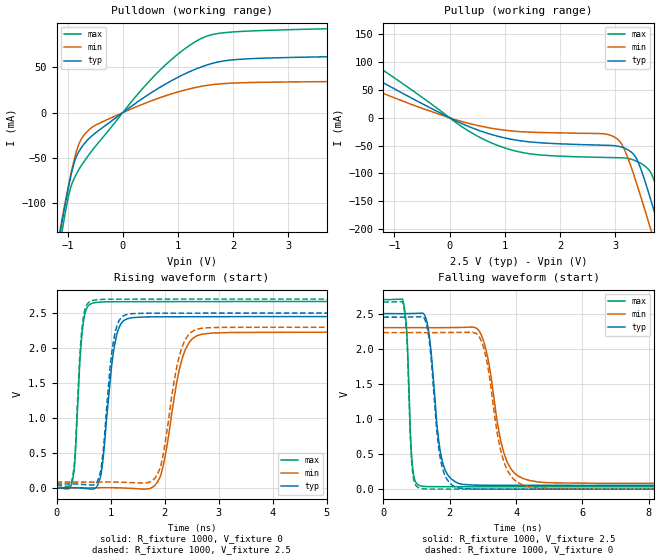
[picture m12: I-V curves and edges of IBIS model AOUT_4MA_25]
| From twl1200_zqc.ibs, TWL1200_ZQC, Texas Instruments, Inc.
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[Model]   AOUT_4MA_25
Model_type  Output
Vref =   2.5
Rref =   1M
Cref =   15p
Vmeas =   1.25
| variable   typ   min   max
C_comp   3.40pF   2.49pF   4.51pF
| C_pullup   3.64pF   2.49pF   4.51pF
| C_pulldown   3.15pF   2.72pF   3.73pF
[Temperature Range]   40   100   -40
| Ambient temperature   25   85   -40
[Voltage range]   2.5   2.3   2.7
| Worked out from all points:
|   slope of the pulldown table from 0 to 0.375 V, typ, clamps not added: 23.1 ohm
|   slope of the pullup table from 0 to 0.375 V, typ, clamps not added: 22.2 ohm
|   rising waveform, R_fixture 1000, V_fixture 0: 20-80 % time 186ps typ, 294ps min, 112ps max; typ from 0 V to 2.45 V
|   falling waveform, R_fixture 1000, V_fixture 2.5: 20-80 % time 289ps typ, 475ps min, 126ps max; typ from 2.5 V to 0.054 V
|   rising waveform, R_fixture 1000, V_fixture 2.5: 20-80 % time 171ps typ, 278ps min, 109ps max; typ from 0.054 V to 2.5 V
|   falling waveform, R_fixture 1000, V_fixture 0: 20-80 % time 278ps typ, 462ps min, 122ps max; typ from 2.45 V to 0 V
[Pulldown]
| AOUT_4MA_25
|   Voltage   I(typ)   I(min)   I(max)
-2.5V     -642.6mA   -610.7mA   -690.5mA
-1.15V    -137.8mA   -133.6mA   -149.9mA
-1.11V    -123.9mA   -120.4mA   -134.9mA
-1.085V   -115.3mA   -112.3mA   -125.8mA
-970mV    -78.33mA   -76.64mA   -88.69mA
-875mV    -54.32mA   -50.76mA   -71.95mA
-770mV    -40.49mA   -31.37mA   -60.2mA
-610mV    -28.5mA    -18.85mA   -46.14mA
575mV     24.18mA    14.3mA     40.68mA
1.41V     50.08mA    28.8mA     81.33mA
2.24V     59.27mA    33.09mA    89.82mA
5V        62.72mA    34.67mA    94.24mA
[Pullup]
| AOUT_4MA_25
|   Voltage   I(typ)   I(min)   I(max)
-2.5V     130mA      93.97mA    163.5mA
-430mV    21.91mA    14.65mA    31.96mA
770mV     -30.37mA   -19.01mA   -45.69mA
1.535V    -44.12mA   -26.1mA    -65.78mA
2.94V     -49.86mA   -32.46mA   -71.64mA
3.125V    -52.97mA   -48.42mA   -72.03mA
3.345V    -66.91mA   -104.7mA   -76.4mA
3.47V     -93.2mA    -143.6mA   -82.2mA
3.64V     -145.6mA   -199.1mA   -97.66mA
3.795V    -198.1mA   -251.1mA   -140.1mA
3.95V     -252.3mA   -304mA     -194.5mA
5V        -635.9mA   -673.3mA   -595.2mA
[Ramp]
| AOUT_4MA_25
| variable   typ   min   max
dV/dt_r   1.48/2.02E-10   1.35/3.05E-10   1.61/1.19E-10
dV/dt_f   1.47/2.94E-10   1.34/4.85E-10   1.60/1.27E-10
R_load = 1000
[Rising Waveform]
| AOUT_4MA_25
R_fixture =   1000
C_fixture =   0
L_fixture =   0
V_fixture =   0
V_fixture_min = 0
V_fixture_max = 0
|   Time   V(typ)   V(min)   V(max)
0s        9.079nV    37.27nV    970.3pV
310ps     1.537mV    -21.75uV   167.8mV
535ps     -9.551mV   -44.8uV    2.52V
820ps     179.2mV    1.28mV     2.657V
970ps     1.341V     1.868mV    2.661V
1.255ns   2.397V     -3.227mV   2.662V
1.92ns    2.446V     163.6mV    2.663V
2.46ns    2.447V     2.086V     2.664V
3.25ns    2.449V     2.222V     2.664V
238.2ns   2.45V      2.23V      2.665V
[Falling Waveform]
| AOUT_4MA_25
R_fixture =   1000
C_fixture =   0
L_fixture =   0
V_fixture =   2.5
V_fixture_min = 2.3
V_fixture_max = 2.7
|   Time   V(typ)   V(min)   V(max)
0s        2.5V       2.3V       2.7V
590ps     2.499V     2.3V       2.686V
705ps     2.5V       2.3V       2.232V
895ps     2.502V     2.3V       247.5mV
1.315ns   2.378V     2.299V     37mV
1.81ns    339mV      2.3V       35.44mV
2.805ns   57.7mV     2.293V     34.71mV
3.77ns    54.88mV    349.4mV    34.46mV
5.225ns   54.27mV    89.05mV    34.33mV
238.2ns   54mV       82.44mV    34.26mV
[Rising Waveform]
| AOUT_4MA_25
R_fixture =   1000
C_fixture =   0
L_fixture =   0
V_fixture =   2.5
V_fixture_min = 2.3
V_fixture_max = 2.7
|   Time   V(typ)   V(min)   V(max)
0s        54mV       82.44mV    34.26mV
300ps     55.39mV    82.42mV    168mV
520ps     45.75mV    82.4mV     2.535V
805ps     209.2mV    83.47mV    2.694V
960ps     1.446V     83.86mV    2.697V
1.23ns    2.457V     79.19mV    2.698V
1.89ns    2.498V     235.1mV    2.699V
2.4ns     2.499V     2.144V     2.699V
3.075ns   2.499V     2.296V     2.7V
238.2ns   2.5V       2.3V       2.7V
[Falling Waveform]
| AOUT_4MA_25
R_fixture =   1000
C_fixture =   0
L_fixture =   0
V_fixture =   0
V_fixture_min = 0
V_fixture_max = 0
|   Time   V(typ)   V(min)   V(max)
0s        2.45V      2.23V      2.665V
590ps     2.45V      2.23V      2.649V
700ps     2.45V      2.23V      2.22V
890ps     2.452V     2.23V      206.4mV
1.325ns   2.295V     2.229V     2.412mV
1.785ns   290.3mV    2.23V      1.052mV
2.69ns    3.516mV    2.234V     452.3uV
3.745ns   752uV      261.4mV    193.3uV
5.115ns   262uV      6.218mV    71.58uV
238.2ns   25.79nV    63.6nV     8.597nV
